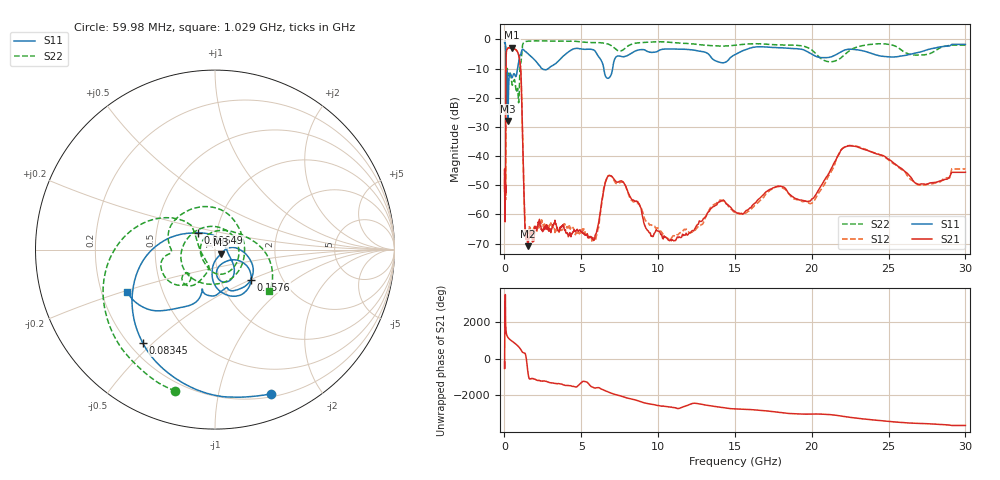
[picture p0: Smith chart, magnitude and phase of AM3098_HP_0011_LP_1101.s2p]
! Date/Time: Thu, Feb 28, 2019 8:34 AM
! Network Analyzer: Agilent Technologies E8364B Rev: A.07.50.67
! Sweep from 0.010 to 30.000 GHz, 1601 Points, Sweep Type: LOG
! Power Supply: 5.023 V, 0.002 A
# Hz S DB R 50
!freq MagS11 AngS11 MagS21 AngS21 MagS12 AngS12 MagS22 AngS22
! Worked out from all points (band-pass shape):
!   1601 points, 10 MHz to 30 GHz, reference 50 ohm
!   highest |S21| = -2.79 dB at 493.1 MHz (marker M1); lowest = -70.9 dB at 1.528 GHz (marker M2)
!   |S21| within 3 dB of the highest: 108.8 MHz to 944.9 MHz (836.1 MHz wide, 159 % of centre)
!   lowest |S11| = -27.9 dB at 233.9 MHz (marker M3), VSWR 1.08, Z = 53.2 - j2.71 ohm
!   |S11| at or under -10 dB: 93.02 MHz to 849.3 MHz (756.2 MHz wide, 161 % of centre); 2.45 GHz to 2.843 GHz (392.3 MHz wide, 14.8 % of centre); 6.467 GHz to 7.041 GHz (574 MHz wide, 8.5 % of centre)
!   |S22| runs from -22.5 to -0.4 dB; largest |S21 - S12| = 0.01
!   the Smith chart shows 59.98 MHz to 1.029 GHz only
!   S11 on the Smith chart (normalised r, x): 59.98 MHz: 0.23, -1.43; 83.45 MHz: 0.25, -0.47; 96.49 MHz: 0.81, +0.16; 157.6 MHz: 1.40, -0.50; 1.029 GHz: 0.31, -0.21
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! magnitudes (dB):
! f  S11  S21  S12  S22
! 10 MHz  -0.3  -44.7  -47.2  -0.6
! 38.04 MHz  -0.5  -60.0  -57.9  -1.0
! 59.98 MHz  -1.3  -51.7  -53.1  -1.7
! 73.27 MHz  -2.0  -51.5  -53.3  -2.5
! 83.45 MHz  -3.6  -36.1  -35.7  -4.0
! 96.49 MHz  -17.5  -11.8  -11.8  -20.9
! 144.7 MHz  -15.4  -3.6  -3.5  -13.0
! 157.6 MHz  -11.6  -3.5  -3.4  -10.9
! 233.9 MHz  -27.9  -2.9  -2.9  -12.1
! 493.1 MHz  -13.1  -2.8  -2.8  -15.5
! 550.5 MHz  -12.4  -3.0  -3.0  -14.9
! 1.029 GHz  -5.3  -8.6  -8.6  -8.4
! 1.328 GHz  -4.0  -63.4  -61.1  -0.8
! 1.528 GHz  -4.9  -70.9  -67.9  -0.6
! 2.084 GHz  -7.7  -65.4  -64.3  -0.4
! 5.754 GHz  -3.5  -68.6  -68.0  -1.1
! 6.719 GHz  -13.3  -47.0  -46.9  -1.5
! 7.926 GHz  -5.7  -50.7  -50.7  -2.7
! 11.03 GHz  -3.3  -69.1  -67.3  -1.1
! 19.8 GHz  -4.5  -55.4  -56.1  -2.9
! 22.67 GHz  -3.4  -36.5  -36.4  -3.2
! 30 GHz  -1.7  -45.5  -44.4  -2.0
